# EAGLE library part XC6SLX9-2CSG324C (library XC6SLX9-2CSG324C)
FPGA - Field Programmable Gate Array XC6SLX9-2CSG324C Source: Datasheet
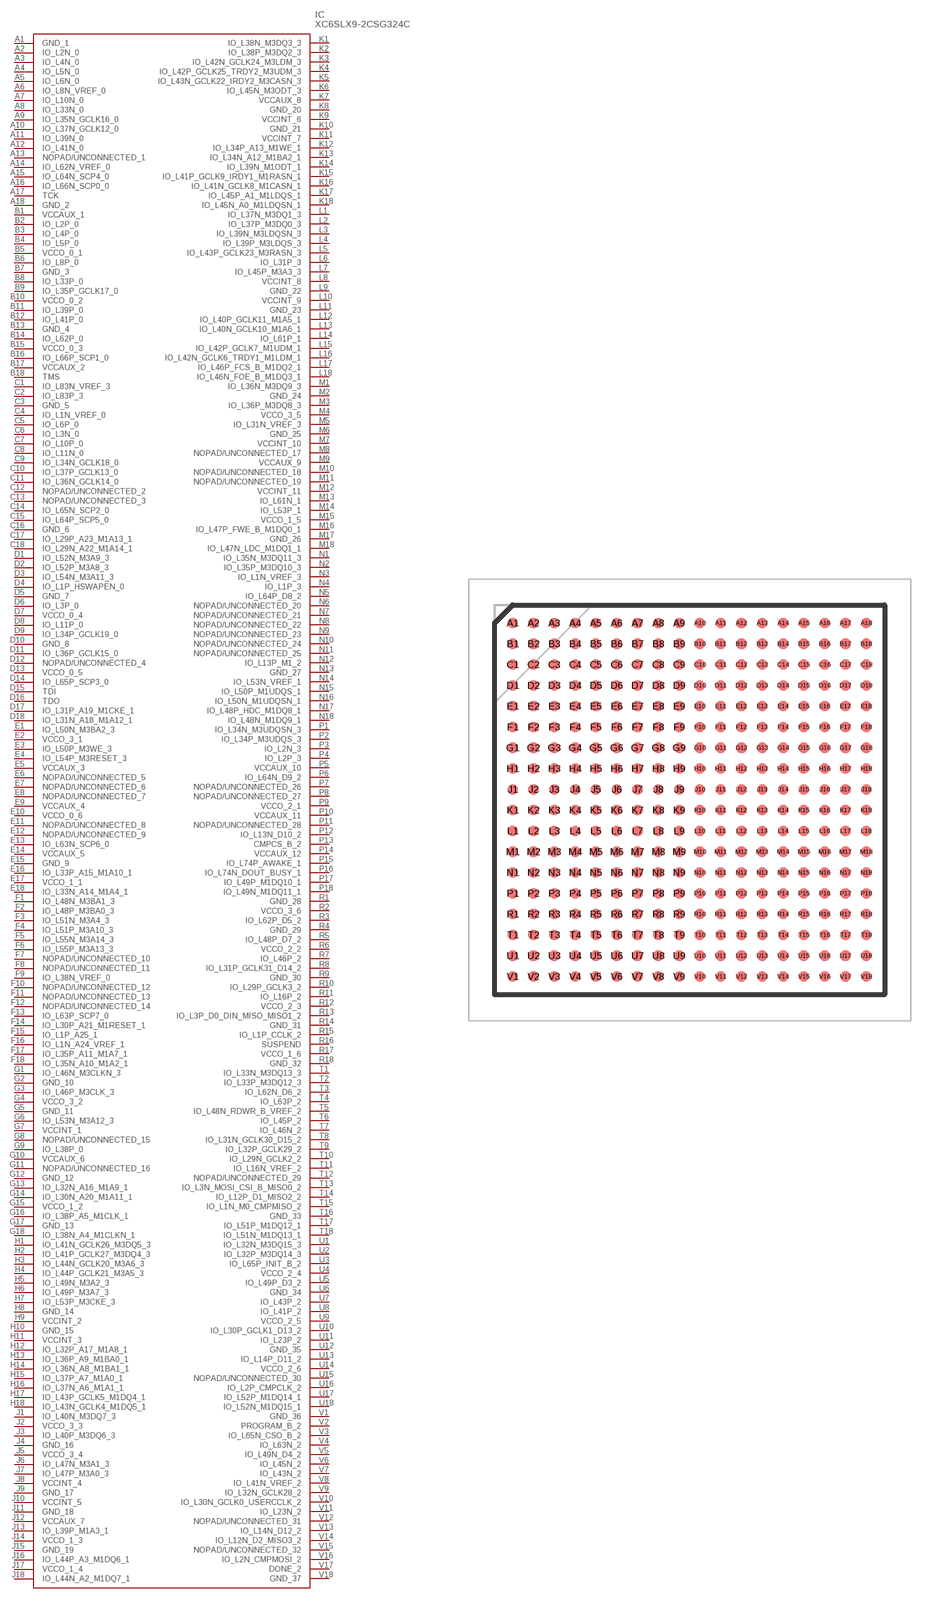
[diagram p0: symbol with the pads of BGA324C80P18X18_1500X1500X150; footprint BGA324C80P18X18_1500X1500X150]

Designator prefix IC

## XC6SLX9-2CSG324C (Description: FPGA - Field Programmable Gate Array XC6SLX9-2CSG324C; Height: 1.5mm; Manufacturer_Name: AMD; Manufacturer_Part_Number: XC6SLX9-2CSG324C; Mouser_Part_Number: 217-XC6SLX9-2CSG324C; Mouser_Price-Stock: https://www.mouser.co.uk/ProductDetail/AMD-Xilinx/XC6SLX9-2CSG324C?qs=rrS6PyfT74dNQmR8a6nohA%3D%3D)  [BGA324C80P18X18_1500X1500X150]
A1  GND_1
A2  IO_L2N_0
A3  IO_L4N_0
A4  IO_L5N_0
A5  IO_L6N_0
A6  IO_L8N_VREF_0
A7  IO_L10N_0
A8  IO_L33N_0
A9  IO_L35N_GCLK16_0
A10  IO_L37N_GCLK12_0
A11  IO_L39N_0
A12  IO_L41N_0
A13  NOPAD/UNCONNECTED_1
A14  IO_L62N_VREF_0
A15  IO_L64N_SCP4_0
A16  IO_L66N_SCP0_0
A17  TCK
A18  GND_2
B1  VCCAUX_1
B2  IO_L2P_0
B3  IO_L4P_0
B4  IO_L5P_0
B5  VCCO_0_1
B6  IO_L8P_0
B7  GND_3
B8  IO_L33P_0
B9  IO_L35P_GCLK17_0
B10  VCCO_0_2
B11  IO_L39P_0
B12  IO_L41P_0
B13  GND_4
B14  IO_L62P_0
B15  VCCO_0_3
B16  IO_L66P_SCP1_0
B17  VCCAUX_2
B18  TMS
C1  IO_L83N_VREF_3
C2  IO_L83P_3
C3  GND_5
C4  IO_L1N_VREF_0
C5  IO_L6P_0
C6  IO_L3N_0
C7  IO_L10P_0
C8  IO_L11N_0
C9  IO_L34N_GCLK18_0
C10  IO_L37P_GCLK13_0
C11  IO_L36N_GCLK14_0
C12  NOPAD/UNCONNECTED_2
C13  NOPAD/UNCONNECTED_3
C14  IO_L65N_SCP2_0
C15  IO_L64P_SCP5_0
C16  GND_6
C17  IO_L29P_A23_M1A13_1
C18  IO_L29N_A22_M1A14_1
D1  IO_L52N_M3A9_3
D2  IO_L52P_M3A8_3
D3  IO_L54N_M3A11_3
D4  IO_L1P_HSWAPEN_0
D5  GND_7
D6  IO_L3P_0
D7  VCCO_0_4
D8  IO_L11P_0
D9  IO_L34P_GCLK19_0
D10  GND_8
D11  IO_L36P_GCLK15_0
D12  NOPAD/UNCONNECTED_4
D13  VCCO_0_5
D14  IO_L65P_SCP3_0
D15  TDI
D16  TDO
D17  IO_L31P_A19_M1CKE_1
D18  IO_L31N_A18_M1A12_1
E1  IO_L50N_M3BA2_3
E2  VCCO_3_1
E3  IO_L50P_M3WE_3
E4  IO_L54P_M3RESET_3
E5  VCCAUX_3
E6  NOPAD/UNCONNECTED_5
E7  NOPAD/UNCONNECTED_6
E8  NOPAD/UNCONNECTED_7
E9  VCCAUX_4
E10  VCCO_0_6
E11  NOPAD/UNCONNECTED_8
E12  NOPAD/UNCONNECTED_9
E13  IO_L63N_SCP6_0
E14  VCCAUX_5
E15  GND_9
E16  IO_L33P_A15_M1A10_1
E17  VCCO_1_1
E18  IO_L33N_A14_M1A4_1
F1  IO_L48N_M3BA1_3
F2  IO_L48P_M3BA0_3
F3  IO_L51N_M3A4_3
F4  IO_L51P_M3A10_3
F5  IO_L55N_M3A14_3
F6  IO_L55P_M3A13_3
F7  NOPAD/UNCONNECTED_10
F8  NOPAD/UNCONNECTED_11
F9  IO_L38N_VREF_0
F10  NOPAD/UNCONNECTED_12
F11  NOPAD/UNCONNECTED_13
F12  NOPAD/UNCONNECTED_14
F13  IO_L63P_SCP7_0
F14  IO_L30P_A21_M1RESET_1
F15  IO_L1P_A25_1
F16  IO_L1N_A24_VREF_1
F17  IO_L35P_A11_M1A7_1
F18  IO_L35N_A10_M1A2_1
G1  IO_L46N_M3CLKN_3
G2  GND_10
G3  IO_L46P_M3CLK_3
G4  VCCO_3_2
G5  GND_11
G6  IO_L53N_M3A12_3
G7  VCCINT_1
G8  NOPAD/UNCONNECTED_15
G9  IO_L38P_0
G10  VCCAUX_6
G11  NOPAD/UNCONNECTED_16
G12  GND_12
G13  IO_L32N_A16_M1A9_1
G14  IO_L30N_A20_M1A11_1
G15  VCCO_1_2
G16  IO_L38P_A5_M1CLK_1
G17  GND_13
G18  IO_L38N_A4_M1CLKN_1
H1  IO_L41N_GCLK26_M3DQ5_3
H2  IO_L41P_GCLK27_M3DQ4_3
H3  IO_L44N_GCLK20_M3A6_3
H4  IO_L44P_GCLK21_M3A5_3
H5  IO_L49N_M3A2_3
H6  IO_L49P_M3A7_3
H7  IO_L53P_M3CKE_3
H8  GND_14
H9  VCCINT_2
H10  GND_15
H11  VCCINT_3
H12  IO_L32P_A17_M1A8_1
H13  IO_L36P_A9_M1BA0_1
H14  IO_L36N_A8_M1BA1_1
H15  IO_L37P_A7_M1A0_1
H16  IO_L37N_A6_M1A1_1
H17  IO_L43P_GCLK5_M1DQ4_1
H18  IO_L43N_GCLK4_M1DQ5_1
J1  IO_L40N_M3DQ7_3
J2  VCCO_3_3
J3  IO_L40P_M3DQ6_3
J4  GND_16
J5  VCCO_3_4
J6  IO_L47N_M3A1_3
J7  IO_L47P_M3A0_3
J8  VCCINT_4
J9  GND_17
J10  VCCINT_5
J11  GND_18
J12  VCCAUX_7
J13  IO_L39P_M1A3_1
J14  VCCO_1_3
J15  GND_19
J16  IO_L44P_A3_M1DQ6_1
J17  VCCO_1_4
J18  IO_L44N_A2_M1DQ7_1
K1  IO_L38N_M3DQ3_3
K2  IO_L38P_M3DQ2_3
K3  IO_L42N_GCLK24_M3LDM_3
K4  IO_L42P_GCLK25_TRDY2_M3UDM_3
K5  IO_L43N_GCLK22_IRDY2_M3CASN_3
K6  IO_L45N_M3ODT_3
K7  VCCAUX_8
K8  GND_20
K9  VCCINT_6
K10  GND_21
K11  VCCINT_7
K12  IO_L34P_A13_M1WE_1
K13  IO_L34N_A12_M1BA2_1
K14  IO_L39N_M1ODT_1
K15  IO_L41P_GCLK9_IRDY1_M1RASN_1
K16  IO_L41N_GCLK8_M1CASN_1
K17  IO_L45P_A1_M1LDQS_1
K18  IO_L45N_A0_M1LDQSN_1
L1  IO_L37N_M3DQ1_3
L2  IO_L37P_M3DQ0_3
L3  IO_L39N_M3LDQSN_3
L4  IO_L39P_M3LDQS_3
L5  IO_L43P_GCLK23_M3RASN_3
L6  IO_L31P_3
L7  IO_L45P_M3A3_3
L8  VCCINT_8
L9  GND_22
L10  VCCINT_9
L11  GND_23
L12  IO_L40P_GCLK11_M1A5_1
L13  IO_L40N_GCLK10_M1A6_1
L14  IO_L61P_1
L15  IO_L42P_GCLK7_M1UDM_1
L16  IO_L42N_GCLK6_TRDY1_M1LDM_1
L17  IO_L46P_FCS_B_M1DQ2_1
L18  IO_L46N_FOE_B_M1DQ3_1
M1  IO_L36N_M3DQ9_3
M2  GND_24
M3  IO_L36P_M3DQ8_3
M4  VCCO_3_5
M5  IO_L31N_VREF_3
M6  GND_25
M7  VCCINT_10
M8  NOPAD/UNCONNECTED_17
M9  VCCAUX_9
M10  NOPAD/UNCONNECTED_18
M11  NOPAD/UNCONNECTED_19
M12  VCCINT_11
M13  IO_L61N_1
M14  IO_L53P_1
M15  VCCO_1_5
M16  IO_L47P_FWE_B_M1DQ0_1
M17  GND_26
M18  IO_L47N_LDC_M1DQ1_1
N1  IO_L35N_M3DQ11_3
N2  IO_L35P_M3DQ10_3
N3  IO_L1N_VREF_3
N4  IO_L1P_3
N5  IO_L64P_D8_2
N6  NOPAD/UNCONNECTED_20
N7  NOPAD/UNCONNECTED_21
N8  NOPAD/UNCONNECTED_22
N9  NOPAD/UNCONNECTED_23
N10  NOPAD/UNCONNECTED_24
N11  NOPAD/UNCONNECTED_25
N12  IO_L13P_M1_2
N13  GND_27
N14  IO_L53N_VREF_1
N15  IO_L50P_M1UDQS_1
N16  IO_L50N_M1UDQSN_1
N17  IO_L48P_HDC_M1DQ8_1
N18  IO_L48N_M1DQ9_1
P1  IO_L34N_M3UDQSN_3
P2  IO_L34P_M3UDQS_3
P3  IO_L2N_3
P4  IO_L2P_3
P5  VCCAUX_10
P6  IO_L64N_D9_2
P7  NOPAD/UNCONNECTED_26
P8  NOPAD/UNCONNECTED_27
P9  VCCO_2_1
P10  VCCAUX_11
P11  NOPAD/UNCONNECTED_28
P12  IO_L13N_D10_2
P13  CMPCS_B_2
P14  VCCAUX_12
P15  IO_L74P_AWAKE_1
P16  IO_L74N_DOUT_BUSY_1
P17  IO_L49P_M1DQ10_1
P18  IO_L49N_M1DQ11_1
R1  GND_28
R2  VCCO_3_6
R3  IO_L62P_D5_2
R4  GND_29
R5  IO_L48P_D7_2
R6  VCCO_2_2
R7  IO_L46P_2
R8  IO_L31P_GCLK31_D14_2
R9  GND_30
R10  IO_L29P_GCLK3_2
R11  IO_L16P_2
R12  VCCO_2_3
R13  IO_L3P_D0_DIN_MISO_MISO1_2
R14  GND_31
R15  IO_L1P_CCLK_2
R16  SUSPEND
R17  VCCO_1_6
R18  GND_32
T1  IO_L33N_M3DQ13_3
T2  IO_L33P_M3DQ12_3
T3  IO_L62N_D6_2
T4  IO_L63P_2
T5  IO_L48N_RDWR_B_VREF_2
T6  IO_L45P_2
T7  IO_L46N_2
T8  IO_L31N_GCLK30_D15_2
T9  IO_L32P_GCLK29_2
T10  IO_L29N_GCLK2_2
T11  IO_L16N_VREF_2
T12  NOPAD/UNCONNECTED_29
T13  IO_L3N_MOSI_CSI_B_MISO0_2
T14  IO_L12P_D1_MISO2_2
T15  IO_L1N_M0_CMPMISO_2
T16  GND_33
T17  IO_L51P_M1DQ12_1
T18  IO_L51N_M1DQ13_1
U1  IO_L32N_M3DQ15_3
U2  IO_L32P_M3DQ14_3
U3  IO_L65P_INIT_B_2
U4  VCCO_2_4
U5  IO_L49P_D3_2
U6  GND_34
U7  IO_L43P_2
U8  IO_L41P_2
U9  VCCO_2_5
U10  IO_L30P_GCLK1_D13_2
U11  IO_L23P_2
U12  GND_35
U13  IO_L14P_D11_2
U14  VCCO_2_6
U15  NOPAD/UNCONNECTED_30
U16  IO_L2P_CMPCLK_2
U17  IO_L52P_M1DQ14_1
U18  IO_L52N_M1DQ15_1
V1  GND_36
V2  PROGRAM_B_2
V3  IO_L65N_CSO_B_2
V4  IO_L63N_2
V5  IO_L49N_D4_2
V6  IO_L45N_2
V7  IO_L43N_2
V8  IO_L41N_VREF_2
V9  IO_L32N_GCLK28_2
V10  IO_L30N_GCLK0_USERCCLK_2
V11  IO_L23N_2
V12  NOPAD/UNCONNECTED_31
V13  IO_L14N_D12_2
V14  IO_L12N_D2_MISO3_2
V15  NOPAD/UNCONNECTED_32
V16  IO_L2N_CMPMOSI_2
V17  DONE_2
V18  GND_37

## Footprint BGA324C80P18X18_1500X1500X150 (pad centres in mm)
(CSG324)
smd 0.41 x 0.41: A1 -6.8,6.8; A2 -6,6.8; A3 -5.2,6.8; A4 -4.4,6.8; A5 -3.6,6.8; A6 -2.8,6.8; A7 -2,6.8; A8 -1.2,6.8; A9 -0.4,6.8; A10 0.4,6.8; A11 1.2,6.8; A12 2,6.8; A13 2.8,6.8; A14 3.6,6.8; A15 4.4,6.8; A16 5.2,6.8; A17 6,6.8; A18 6.8,6.8; B1 -6.8,6; B2 -6,6; B3 -5.2,6; B4 -4.4,6; B5 -3.6,6; B6 -2.8,6; B7 -2,6; B8 -1.2,6; B9 -0.4,6; B10 0.4,6; B11 1.2,6; B12 2,6; B13 2.8,6; B14 3.6,6; B15 4.4,6; B16 5.2,6; B17 6,6; B18 6.8,6; C1 -6.8,5.2; C2 -6,5.2; C3 -5.2,5.2; C4 -4.4,5.2; C5 -3.6,5.2; C6 -2.8,5.2; C7 -2,5.2; C8 -1.2,5.2; C9 -0.4,5.2; C10 0.4,5.2; C11 1.2,5.2; C12 2,5.2; C13 2.8,5.2; C14 3.6,5.2; C15 4.4,5.2; C16 5.2,5.2; C17 6,5.2; C18 6.8,5.2; D1 -6.8,4.4; D2 -6,4.4; D3 -5.2,4.4; D4 -4.4,4.4; D5 -3.6,4.4; D6 -2.8,4.4; D7 -2,4.4; D8 -1.2,4.4; D9 -0.4,4.4; D10 0.4,4.4; D11 1.2,4.4; D12 2,4.4; D13 2.8,4.4; D14 3.6,4.4; D15 4.4,4.4; D16 5.2,4.4; D17 6,4.4; D18 6.8,4.4; E1 -6.8,3.6; E2 -6,3.6; E3 -5.2,3.6; E4 -4.4,3.6; E5 -3.6,3.6; E6 -2.8,3.6; E7 -2,3.6; E8 -1.2,3.6; E9 -0.4,3.6; E10 0.4,3.6; E11 1.2,3.6; E12 2,3.6; E13 2.8,3.6; E14 3.6,3.6; E15 4.4,3.6; E16 5.2,3.6; E17 6,3.6; E18 6.8,3.6; F1 -6.8,2.8; F2 -6,2.8; F3 -5.2,2.8; F4 -4.4,2.8; F5 -3.6,2.8; F6 -2.8,2.8; F7 -2,2.8; F8 -1.2,2.8; F9 -0.4,2.8; F10 0.4,2.8; F11 1.2,2.8; F12 2,2.8; F13 2.8,2.8; F14 3.6,2.8; F15 4.4,2.8; F16 5.2,2.8; F17 6,2.8; F18 6.8,2.8; G1 -6.8,2; G2 -6,2; G3 -5.2,2; G4 -4.4,2; G5 -3.6,2; G6 -2.8,2; G7 -2,2; G8 -1.2,2; G9 -0.4,2; G10 0.4,2; G11 1.2,2; G12 2,2; G13 2.8,2; G14 3.6,2; G15 4.4,2; G16 5.2,2; G17 6,2; G18 6.8,2; H1 -6.8,1.2; H2 -6,1.2; H3 -5.2,1.2; H4 -4.4,1.2; H5 -3.6,1.2; H6 -2.8,1.2; H7 -2,1.2; H8 -1.2,1.2; H9 -0.4,1.2; H10 0.4,1.2; H11 1.2,1.2; H12 2,1.2; H13 2.8,1.2; H14 3.6,1.2; H15 4.4,1.2; H16 5.2,1.2; H17 6,1.2; H18 6.8,1.2; J1 -6.8,0.4; J2 -6,0.4; J3 -5.2,0.4; J4 -4.4,0.4; J5 -3.6,0.4; J6 -2.8,0.4; J7 -2,0.4; J8 -1.2,0.4; J9 -0.4,0.4; J10 0.4,0.4; J11 1.2,0.4; J12 2,0.4; J13 2.8,0.4; J14 3.6,0.4; J15 4.4,0.4; J16 5.2,0.4; J17 6,0.4; J18 6.8,0.4; K1 -6.8,-0.4; K2 -6,-0.4; K3 -5.2,-0.4; K4 -4.4,-0.4; K5 -3.6,-0.4; K6 -2.8,-0.4; K7 -2,-0.4; K8 -1.2,-0.4; K9 -0.4,-0.4; K10 0.4,-0.4; K11 1.2,-0.4; K12 2,-0.4; K13 2.8,-0.4; K14 3.6,-0.4; K15 4.4,-0.4; K16 5.2,-0.4; K17 6,-0.4; K18 6.8,-0.4; L1 -6.8,-1.2; L2 -6,-1.2; L3 -5.2,-1.2; L4 -4.4,-1.2; L5 -3.6,-1.2; L6 -2.8,-1.2; L7 -2,-1.2; L8 -1.2,-1.2; L9 -0.4,-1.2; L10 0.4,-1.2; L11 1.2,-1.2; L12 2,-1.2; L13 2.8,-1.2; L14 3.6,-1.2; L15 4.4,-1.2; L16 5.2,-1.2; L17 6,-1.2; L18 6.8,-1.2; M1 -6.8,-2; M2 -6,-2; M3 -5.2,-2; M4 -4.4,-2; M5 -3.6,-2; M6 -2.8,-2; M7 -2,-2; M8 -1.2,-2; M9 -0.4,-2; M10 0.4,-2; M11 1.2,-2; M12 2,-2; M13 2.8,-2; M14 3.6,-2; M15 4.4,-2; M16 5.2,-2; M17 6,-2; M18 6.8,-2; N1 -6.8,-2.8; N2 -6,-2.8; N3 -5.2,-2.8; N4 -4.4,-2.8; N5 -3.6,-2.8; N6 -2.8,-2.8; N7 -2,-2.8; N8 -1.2,-2.8; N9 -0.4,-2.8; N10 0.4,-2.8; N11 1.2,-2.8; N12 2,-2.8; N13 2.8,-2.8; N14 3.6,-2.8; N15 4.4,-2.8; N16 5.2,-2.8; N17 6,-2.8; N18 6.8,-2.8; P1 -6.8,-3.6; P2 -6,-3.6; P3 -5.2,-3.6; P4 -4.4,-3.6; P5 -3.6,-3.6; P6 -2.8,-3.6; P7 -2,-3.6; P8 -1.2,-3.6; P9 -0.4,-3.6; P10 0.4,-3.6; P11 1.2,-3.6; P12 2,-3.6; P13 2.8,-3.6; P14 3.6,-3.6; P15 4.4,-3.6; P16 5.2,-3.6; P17 6,-3.6; P18 6.8,-3.6; R1 -6.8,-4.4; R2 -6,-4.4; R3 -5.2,-4.4; R4 -4.4,-4.4; R5 -3.6,-4.4; R6 -2.8,-4.4; R7 -2,-4.4; R8 -1.2,-4.4; R9 -0.4,-4.4; R10 0.4,-4.4; R11 1.2,-4.4; R12 2,-4.4; R13 2.8,-4.4; R14 3.6,-4.4; R15 4.4,-4.4; R16 5.2,-4.4; R17 6,-4.4; R18 6.8,-4.4; T1 -6.8,-5.2; T2 -6,-5.2; T3 -5.2,-5.2; T4 -4.4,-5.2; T5 -3.6,-5.2; T6 -2.8,-5.2; T7 -2,-5.2; T8 -1.2,-5.2; T9 -0.4,-5.2; T10 0.4,-5.2; T11 1.2,-5.2; T12 2,-5.2; T13 2.8,-5.2; T14 3.6,-5.2; T15 4.4,-5.2; T16 5.2,-5.2; T17 6,-5.2; T18 6.8,-5.2; U1 -6.8,-6; U2 -6,-6; U3 -5.2,-6; U4 -4.4,-6; U5 -3.6,-6; U6 -2.8,-6; U7 -2,-6; U8 -1.2,-6; U9 -0.4,-6; U10 0.4,-6; U11 1.2,-6; U12 2,-6; U13 2.8,-6; U14 3.6,-6; U15 4.4,-6; U16 5.2,-6; U17 6,-6; U18 6.8,-6; V1 -6.8,-6.8; V2 -6,-6.8; V3 -5.2,-6.8; V4 -4.4,-6.8; V5 -3.6,-6.8; V6 -2.8,-6.8; V7 -2,-6.8; V8 -1.2,-6.8; V9 -0.4,-6.8; V10 0.4,-6.8; V11 1.2,-6.8; V12 2,-6.8; V13 2.8,-6.8; V14 3.6,-6.8; V15 4.4,-6.8; V16 5.2,-6.8; V17 6,-6.8; V18 6.8,-6.8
